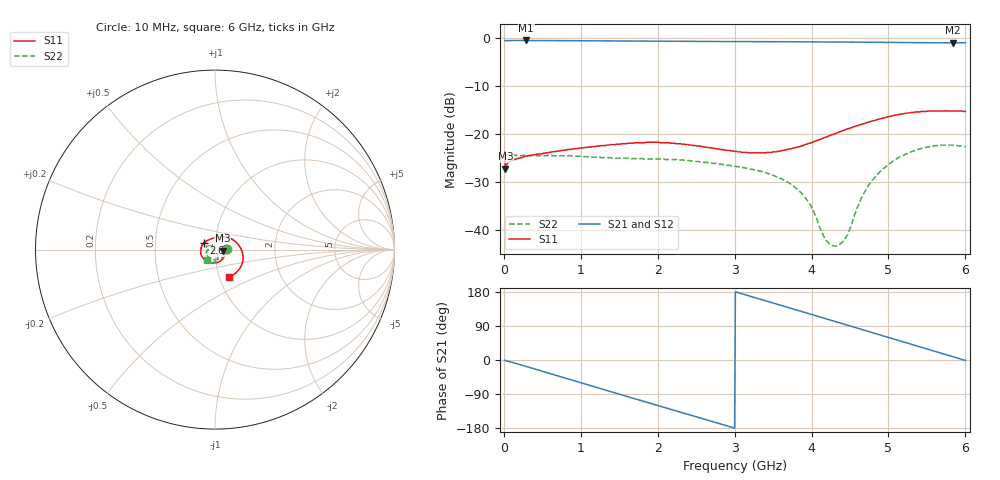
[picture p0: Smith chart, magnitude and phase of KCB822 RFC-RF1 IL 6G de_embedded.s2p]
! "!Agilent Technologies,N5230A,MY45001650,A.07.50.48"
!Agilent	N5230A:	A.07.50.48
! "!Date: Wednesday, February 12, 2014 15:15:43"
! "!Correction: S11(Full 2 Port(1,2)) "
! "!S21(Full 2 Port(1,2)) "
! "!S12(Full 2 Port(1,2)) "
! "!S22(Full 2 Port(1,2)) "
! "!S2P File: Measurements: S11, S21, S12, S22:"
#	Hz	S	dB	R	50
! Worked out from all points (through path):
!   600 points, 10 MHz to 6 GHz, reference 50 ohm
!   highest |S21| = -0.55 dB at 290 MHz (marker M1); lowest = -1.0 dB at 5.84 GHz (marker M2)
!   group delay of S21, straight-line fit = 167 ps
!   lowest |S11| = -27.2 dB at 20 MHz (marker M3), VSWR 1.09, Z = 54.5 - j0.618 ohm
!   |S11| at or under -10 dB: start of sweep to end of sweep
!   |S22| runs from -43.3 to -22.3 dB; largest |S21 - S12| = 0.016
!   S11 on the Smith chart (normalised r, x): 10 MHz: 1.13, +0.01; 2.68 GHz: 0.88, +0.06; 6 GHz: 1.11, -0.35
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1e7  -24.20 2.7  -0.55 -0.7  -0.55 -0.9  -23.60 5.1
2e7  -27.20 -7.5  -0.59 -1.3  -0.59 -1.3  -25.00 -2.4
2.9e8  -24.60 -16.8  -0.55 -16.9  -0.55 -16.9  -24.50 -10.6
6.4e8  -23.70 -42.3  -0.58 -38.2  -0.58 -38.2  -24.50 -29.0
1.01e9  -22.90 -73.6  -0.61 -60.5  -0.61 -60.5  -24.60 -52.7
1.51e9  -22.10 -119.0  -0.66 -90.7  -0.66 -90.7  -25.00 -91.3
2.01e9  -21.70 -161.0  -0.71 -121.0  -0.71 -121.0  -25.20 -128.0
2.33e9  -22.10 175.0  -0.74 -140.0  -0.74 -140.0  -25.40 -147.0
2.68e9  -22.80 151.0  -0.76 -161.0  -0.76 -161.0  -26.00 -161.0
3.01e9  -23.60 130.0  -0.78 180.0  -0.78 180.0  -26.70 -169.0
3.31e9  -23.90 111.0  -0.80 162.0  -0.80 162.0  -27.60 -176.0
3.66e9  -23.30 86.1  -0.81 141.0  -0.81 141.0  -29.70 174.0
3.87e9  -22.50 71.0  -0.83 128.0  -0.83 128.0  -32.30 168.0
4.01e9  -21.70 61.0  -0.85 120.0  -0.85 120.0  -35.50 164.0
4.19e9  -20.60 48.4  -0.86 109.0  -0.86 109.0  -42.10 -162.0
4.35e9  -19.60 37.5  -0.87 99.0  -0.87 99.0  -43.10 -112.0
4.46e9  -19.00 30.1  -0.88 92.3  -0.88 92.3  -41.10 -77.1
4.72e9  -17.60 13.1  -0.91 76.5  -0.91 76.5  -31.20 -59.1
5.01e9  -16.40 -5.1  -0.95 58.9  -0.95 58.9  -26.20 -72.2
5.43e9  -15.30 -30.2  -1.01 33.4  -1.01 33.4  -23.00 -95.1
5.84e9  -15.20 -53.7  -1.04 8.6  -1.04 8.6  -22.30 -119.0
6e9  -15.30 -63.0  -1.03 -1.1  -1.03 -1.1  -22.70 -128.0
